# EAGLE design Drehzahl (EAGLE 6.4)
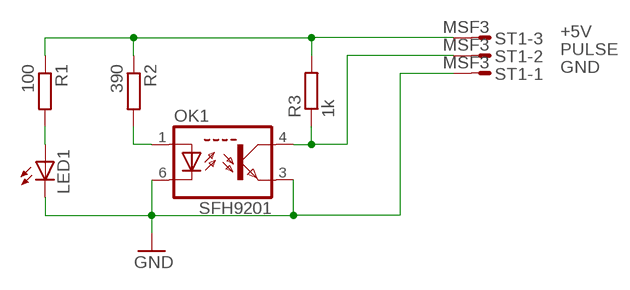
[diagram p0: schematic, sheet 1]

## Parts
LED1  LED3MM  [LED3MM]
OK1  SFH9201  [SO06]
R1  100  R-EU_R0805  [R0805]
R2  390  R-EU_R0805  [R0805]
R3  1k  R-EU_R0805  [R0805]
ST1  MSF3  [MSF3]

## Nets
+5V: R1.1 R2.1 R3.2 ST1.3
GND: LED1.K(C) OK1.3(TE) OK1.6(DC) ST1.1
N$1: OK1.1(DA) R2.2
N$5: LED1.A R1.2
PULSE: OK1.4(TC) R3.1 ST1.2

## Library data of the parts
LED1 = led:LED: LED
OK1 = sfh920x:SFH9201
R1-R3 = rcl:R-EU_: RESISTOR, European symbol
ST1 = con-lumberg:MSF3: MSF CONNECTOR; OC_FARNELL: unknown; OC_NEWARK: unknown

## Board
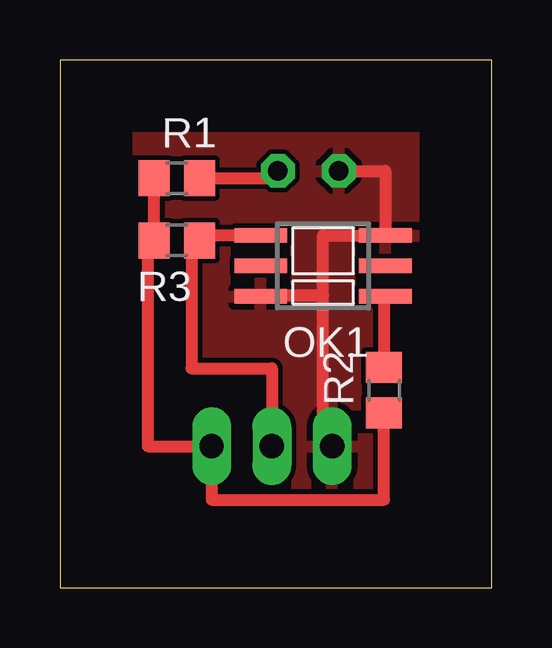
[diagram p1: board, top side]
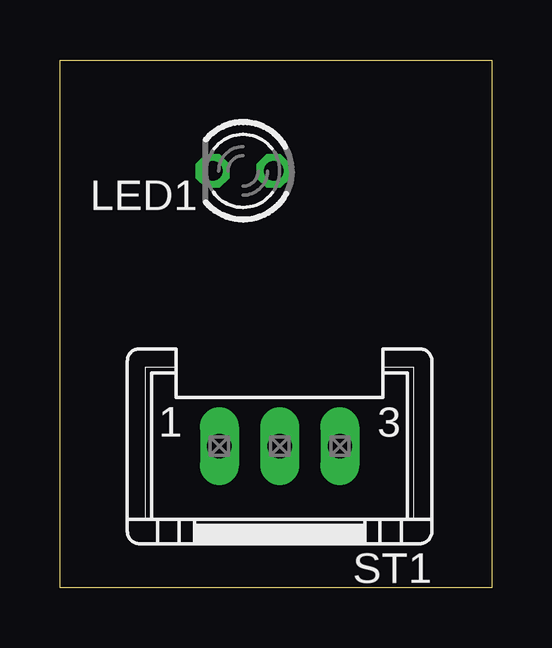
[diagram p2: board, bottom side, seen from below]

Size 18 x 22 mm. Coordinates in mm from the lower left corner, seen from the top.
Outline: 0,0 18,0 18,22 0,22 0,0
Copper layers (1*16): Top 0.035559375mm / dielectric 1.501140625mm / Bottom 0.035559375mm
Design rules "designrules": minimum track width 0.29971875mm, minimum drill 24mil, track to track 0.200659375mm, track to pad 0.200659375mm, pad to pad 0.200659375mm, via to via 0.200659375mm, smd to smd 0.200659375mm, copper to edge 2.999740625mm, drill to drill 8mil, minimum pad ring 0.29971875mm, minimum via ring 0.29971875mm, stop-mask expansion 4mil, vias tented up to drill 0mil, thermal gap 10mil

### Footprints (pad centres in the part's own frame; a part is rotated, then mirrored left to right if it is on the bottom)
LED3MM = drill 0.813 octagon: A -1.27,0; K 1.27,0
SO06 = smd 0.6 x 2.2: 1 -1.27,-2.6; 2 0,-2.6; 3 1.27,-2.6; 4 1.27,2.6; 5 0,2.6; 6 -1.27,2.6
R0805 = smd 1.3 x 1.5: 1 -0.95,0; 2 0.95,0
MSF3 = drill 1.016 long: 1 2.515,-2.54; 2 0,-2.54; 3 -2.515,-2.54

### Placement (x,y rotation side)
LED1  10.36,17.37 180 bottom
OK1  10.97,13.41 90 top
R1  4.88,17.07 0 top
R2  13.51,8.23 90 top
R3  4.88,14.48 180 top
ST1  8.84,3.35 180 bottom

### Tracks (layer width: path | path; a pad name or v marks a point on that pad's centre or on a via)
+5V
  Top 0.406: 3.56,14.48 R3.2 3.66,14.48
  Top 0.5: R3.2 R1.1 | 3.66,14.48 3.66,5.89 ST1.3 6.33,3.66 13.51,3.66 R2.1
GND
  Top 0.406: 8.64,12.14 OK1.6 8.37,12.19
  Top 0.5: 8.37,12.19 10.97,12.19 | 10.97,12.19 10.97,14.68 OK1.3 13.57,17.37 LED1.K | ST1.1 10.97,5.89 10.97,12.19
  pour Top: 0.3,21.64 17.68,21.64 17.68,0.3 0.3,0.3
N$1
  Top 0.406: OK1.1 13.51,12.14
  Top 0.5: 13.51,12.14 R2.2
N$5
  Top 0.5: R1.2 9.09,17.07 LED1.A
PULSE
  Top 0.406: 6.1,14.48 R3.1 | 5.52,14.68 R3.1 | R3.1 5.49,14.48
  Top 0.5: OK1.4 5.52,14.68 | 5.49,14.48 5.49,9.14 8.84,9.14 ST1.2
